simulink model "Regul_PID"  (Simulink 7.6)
settings: Solver=ode5  StartTime=0.0  StopTime=100  RelTol=1e-3
InitFcn:
  | Ts=1;
StopFcn:
  | close all, clc
  | 
  | load csg_sortie.mat
  | plot(x(1,:),x(2,:), x(1,:),x(3,:))
  | grid
  | title('Signaux de consigne et de sortie')
  | xlabel('temps')
  | axis([0 100 0 1.2])
  | 
  | figure
  | load err_cmde.mat
  | plotyy(y(1,:),y(2,:), y(1,:), y(3,:))
  | grid
  | title('Signaux d''erreur et de commande')
  | xlabel('temps')
  | 
  | delete *.mat, clear all
libraries: powerlib_extras x2

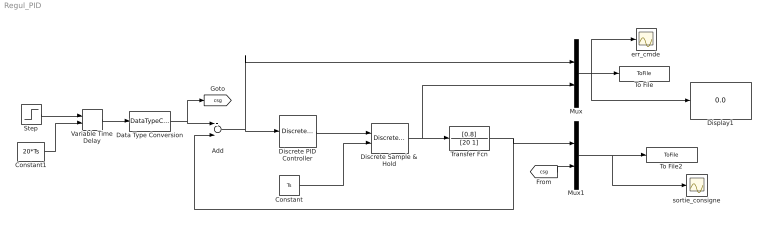
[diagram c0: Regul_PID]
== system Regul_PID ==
  Add : Sum  Inputs=+-
  Constant : Constant  Value=Ts
  Constant1 : Constant  Value=20*Ts
  Data Type Conversion : DataTypeConversion  OutDataTypeStr=double
  Discrete PID Controller : powerlib_extras/Discrete  Control Blocks/Discrete PID Controller  DialogController=POWERSYS.PowerSysDialog  SystemSampleTime=-1  Kp=5  Ki=0.5  Kd=0.01  TcD=1  Par_Limits=[100 -100]  Init=0  Ts=Ts
  Discrete Sample & Hold : powerlib_extras/Discrete  Control Blocks/Discrete Sample & Hold  DialogController=POWERSYS.PowerSysDialog  SystemSampleTime=-1  ic=0  Ts=Ts
  Display1 : Display
  Mux : Mux  Inputs=2
  Mux1 : Mux  Inputs=2
  Step : Step  SampleTime=0
  To File : ToFile  Filename=err_cmde  MatrixName=y
  To File2 : ToFile  Filename=csg_sortie  MatrixName=x
  Transfer Fcn : TransferFcn  Numerator=[0.8]  Denominator=[20 1]
  Variable Time Delay : VariableTransportDelay  MaximumDelay=10
  err_cmde : Scope
  sortie_consigne : Scope
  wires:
  Add/1 -> Discrete PID Controller/1, Mux/1
  Discrete PID Controller/1 -> Discrete Sample & Hold/1
  Discrete Sample & Hold/1 -> Transfer Fcn/1, Mux/2
  Transfer Fcn/1 -> Add/2, Mux1/1
  Constant/1 -> Discrete Sample & Hold/2
  Mux/1 -> To File/1, err_cmde/1, Display1/1
  Mux1/1 -> To File2/1, sortie_consigne/1
  [csg] -> Mux1/2
  Data Type Conversion/1 -> Add/1, [csg]
  Variable Time Delay/1 -> Data Type Conversion/1
  Step/1 -> Variable Time Delay/1
  Constant1/1 -> Variable Time Delay/2
